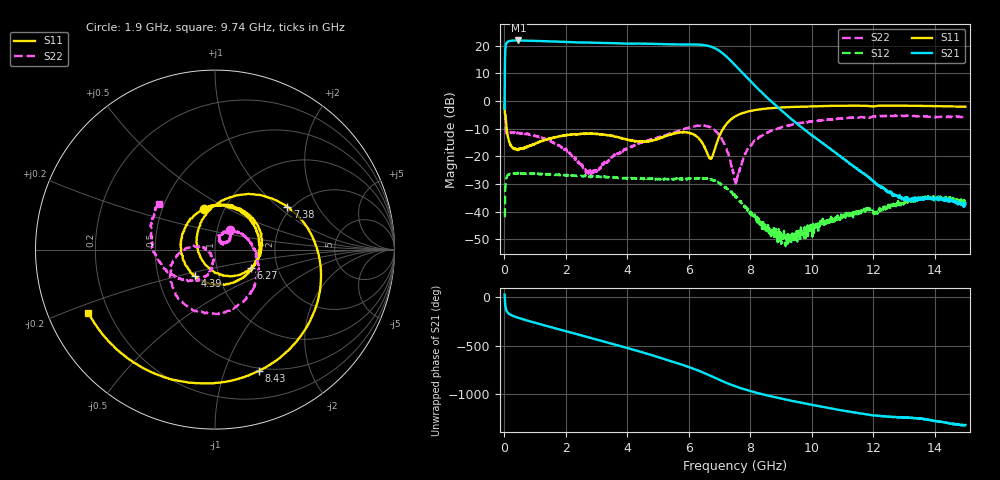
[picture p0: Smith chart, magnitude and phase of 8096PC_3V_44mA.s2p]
!Keysight Technologies,N5247B,US58420632,A.15.75.19
!Date: Wednesday, November 02, 2022 15:45:29
!Correction: S11(C  2-Port  )
!S21(C  2-Port  )
!S12(C  2-Port  )
!S22(C  2-Port  )
!S2P File: Measurements: S11, S21, S12, S22:
# Hz S  dB  R 50
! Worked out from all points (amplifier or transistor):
!   1500 points, 10 MHz to 15 GHz, reference 50 ohm
!   highest |S21| = 21.8 dB at 460 MHz (marker M1)
!   |S21| within 3 dB of that: 35.54 MHz to 6.879 GHz (6.844 GHz wide, 198 % of centre)
!   unconditionally stable (mu >= 1): 11.58 MHz to end of sweep
!   at 2.51 GHz: K = 1.17, MAG = 21.6 dB, |S12| = -27.1 dB
!   at 7.51 GHz: K = 4.31, MAG = 14.4 dB, |S12| = -34.4 dB
!   at 15 GHz: K = 625.87, MAG = -31.3 dB, |S12| = -36.2 dB
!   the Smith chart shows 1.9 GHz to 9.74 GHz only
!   S11 on the Smith chart (normalised r, x): 1.9 GHz: 0.80, +0.38; 4.39 GHz: 0.77, -0.23; 6.27 GHz: 1.47, -0.31; 7.38 GHz: 1.88, +1.15; 8.43 GHz: 0.47, -1.31; 9.74 GHz: 0.12, -0.23
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1e7  -1.59 -33.5  -2.86 28.5  -41.41 -134.9  -0.17 -36.2
1e8  -11.75 -113.8  21.28 -153.5  -26.96 44.9  -11.69 -140.8
1.5e8  -14.47 -129.0  21.58 -169.1  -26.58 23.6  -11.54 -156.1
4.6e8  -17.60 -162.5  21.84 148.1  -25.90 -23.0  -11.63 159.1
1.13e9  -14.91 157.4  21.65 86.4  -26.32 -78.5  -12.96 103.2
1.9e9  -12.67 105.7  21.35 19.7  -26.75 -135.7  -17.09 52.4
2.51e9  -11.80 62.0  21.10 -32.3  -27.15 177.4  -23.03 32.6
3.36e9  -12.40 -9.7  20.92 -105.9  -27.41 113.5  -21.75 71.7
3.89e9  -13.66 -63.9  20.71 -152.9  -27.78 73.5  -17.73 51.9
4.39e9  -14.72 -127.2  20.70 162.4  -28.04 33.8  -15.27 30.2
5.01e9  -13.58 141.6  20.56 103.6  -28.13 -17.8  -13.11 0.6
5.75e9  -11.32 44.2  20.41 29.2  -27.93 -81.8  -10.48 -42.9
6.27e9  -12.93 -26.4  20.34 -29.4  -27.89 -131.8  -8.93 -84.0
6.73e9  -20.76 -166.8  19.56 -91.1  -28.34 174.3  -9.78 -132.8
7.05e9  -11.42 83.8  17.66 -137.6  -30.20 135.5  -13.28 -171.1
7.38e9  -6.59 30.7  14.38 178.8  -32.83 99.1  -22.92 171.5
7.51e9  -5.58 14.4  12.92 163.6  -34.41 86.7  -28.32 -159.6
8.43e9  -2.87 -70.1  2.52 78.4  -45.22 37.6  -12.19 -137.0
9.74e9  -2.04 -153.5  -10.17 -10.9  -47.96 48.4  -7.93 140.5
1.001e10  -1.96 -168.6  -12.38 -27.5  -46.22 37.3  -7.24 125.0
1.251e10  -1.70 61.8  -32.77 -148.2  -37.69 -78.5  -5.38 -10.3
1.5e10  -2.06 -65.7  -36.94 125.5  -36.21 133.3  -5.69 -147.7
